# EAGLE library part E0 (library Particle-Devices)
Particle’s E Series module platform is the World’s simplest solution for developing and deploying cellular-connected IoT products. Product Page : Datasheet Github : Particle devices library
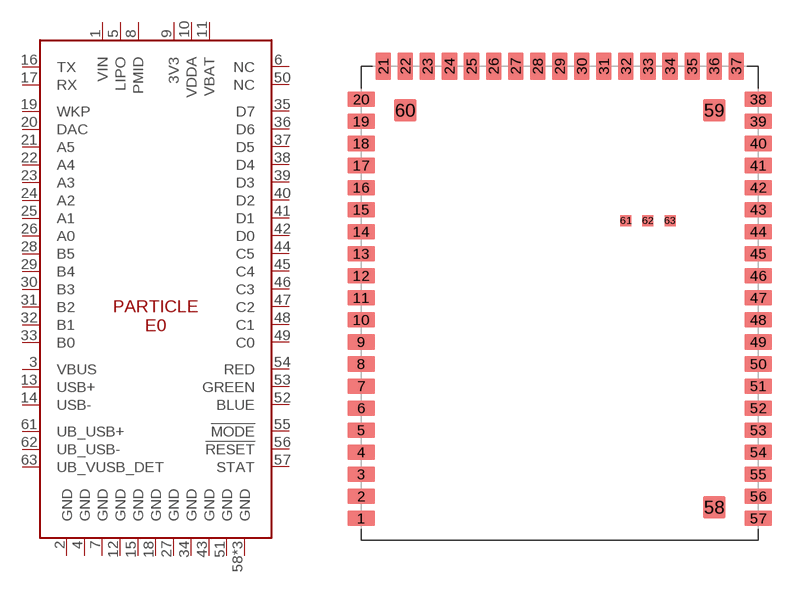
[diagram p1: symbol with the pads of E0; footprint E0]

Designator prefix U

## E0_V005  [E0]
1  VIN
2  GND
3  VBUS
4  GND
5  LIPO
6  NC
7  GND
8  PMID
9  3V3
10  VDDA
11  VBAT
12  GND
13  USB+
14  USB-
15  GND
16  TX
17  RX
18  GND
19  WKP
20  DAC
21  A5
22  A4
23  A3
24  A2
25  A1
26  A0
27  GND
28  B5
29  B4
30  B3
31  B2
32  B1
33  B0
34  GND
35  D7
36  D6
37  D5
38  D4
39  D3
40  D2
41  D1
42  D0
43  GND
44  C5
45  C4
46  C3
47  C2
48  C1
49  C0
50  NC
51  GND
52  BLUE
53  GREEN
54  RED
55  !MODE
56  !RESET
57  STAT
58  GND
59  GND
60  GND
61  UB_USB+
62  UB_USB-
63  UB_VUSB_DET

## Footprint E0 (pad centres in mm)
smd 2.5 x 1.4: 1 -0.008,2; 2 -0.008,4; 3 -0.008,6; 4 -0.008,8; 5 -0.008,10; 6 -0.008,12; 7 -0.008,14; 8 -0.008,16; 9 -0.008,18; 10 -0.008,20; 11 -0.008,22; 12 -0.008,24; 13 -0.008,26; 14 -0.008,28; 15 -0.008,30; 16 -0.008,32; 17 -0.008,34; 18 -0.008,36; 19 -0.008,38; 20 -0.008,40; 38 36.008,40; 39 36.008,38; 40 36.008,36; 41 36.008,34; 42 36.008,32; 43 36.008,30; 44 36.008,28; 45 36.008,26; 46 36.008,24; 47 36.008,22; 48 36.008,20; 49 36.008,18; 50 36.008,16; 51 36.008,14; 52 36.008,12; 53 36.008,10; 54 36.008,8; 55 36.008,6; 56 36.008,4; 57 36.008,2
smd 1.4 x 2.5: 21 2,43.008; 22 4,43.008; 23 6,43.008; 24 8,43.008; 25 10,43.008; 26 12,43.008; 27 14,43.008; 28 16,43.008; 29 18,43.008; 30 20,43.008; 31 22,43.008; 32 24,43.008; 33 26,43.008; 34 28,43.008; 35 30,43.008; 36 32,43.008; 37 34,43.008
smd 2 x 2: 58 32,3; 59 32,39; 60 4,39
smd 1 x 1: 61 24,29; 62 26,29; 63 28,29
